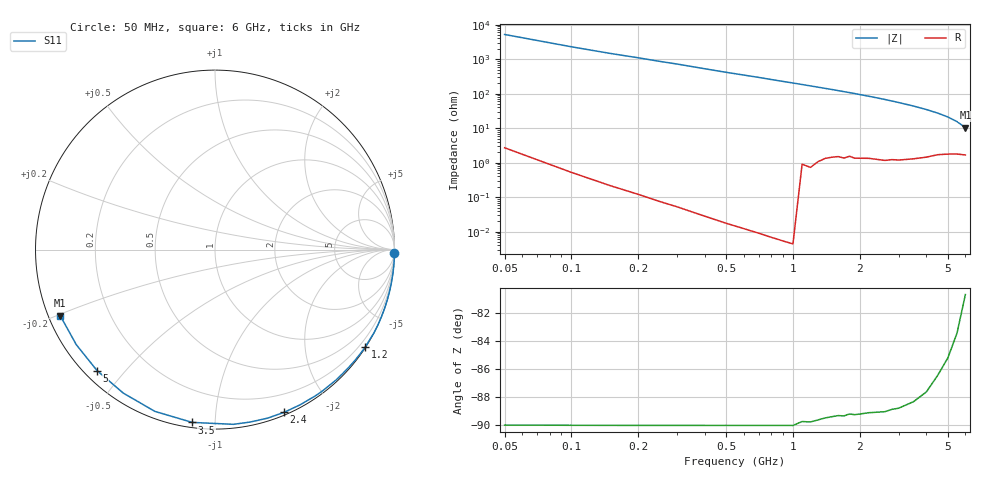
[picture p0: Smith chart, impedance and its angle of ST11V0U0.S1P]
! SIEMENS Discrete & RF Semiconductors
! BA892
! Si PIN Diode in SCD-80
! VR = 11 V
! S-Parameters:  September  1997
# GHz  S  MA  R  50
!  f  S11
! GHz  MAG  ANG
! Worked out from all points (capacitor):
!   34 points, 50 MHz to 6 GHz, reference 50 ohm
!   read as one part to ground: C = 695 fF near 50 MHz
!   lowest |Z| = 10.3 ohm at 6 GHz (marker M1)
!   S11 on the Smith chart (normalised r, x): 50 MHz: open; 1.2 GHz: 0.01, -3.37; 2.4 GHz: 0.02, -1.51; 3.5 GHz: 0.03, -0.88; 5 GHz: 0.04, -0.42; 6 GHz: 0.03, -0.20
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0.05  1 -1.1
0.2  1 -5.2
0.3  1 -7.9
0.4  1 -10.8
0.5  1 -13.7
0.6  1 -16.4
0.7  1 -19.1
0.8  1 -22.0
0.9  1 -24.8
1  1 -27.5
1.2  0.9976 -33.1
1.4  0.9941 -38.7
1.5  0.9928 -41.4
1.6  0.9915 -44.3
1.7  0.9913 -47.1
1.9  0.9894 -52.7
2  0.9883 -55.6
2.2  0.9862 -61.3
2.4  0.9849 -67.0
2.6  0.9838 -72.7
2.8  0.9805 -78.4
3  0.9788 -84.0
3.5  0.9711 -97.5
4  0.9616 -110.4
4.5  0.9488 -122.6
5  0.9415 -134.2
5.5  0.9369 -145.6
6  0.9376 -156.9
